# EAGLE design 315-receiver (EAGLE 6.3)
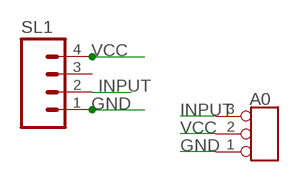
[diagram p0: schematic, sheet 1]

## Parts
A0  TINKER_3P_DIP  [3P_2.0_DIP]
SL1  M04  [4P-NEW]

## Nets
GND: A0.1 SL1.1
INPUT: A0.3 SL1.2
VCC: A0.2 SL1.4
Unconnected: SL1.3

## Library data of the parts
A0 = Connector:TINKER_3P_DIP
SL1 = con-amp-quick:M04: AMP QUICK CONNECTOR

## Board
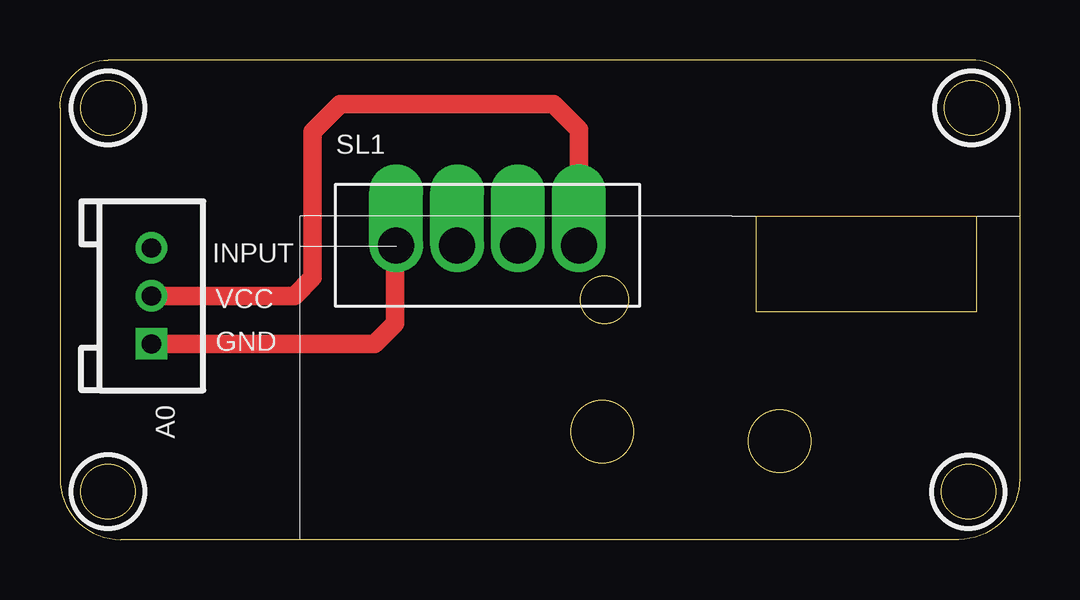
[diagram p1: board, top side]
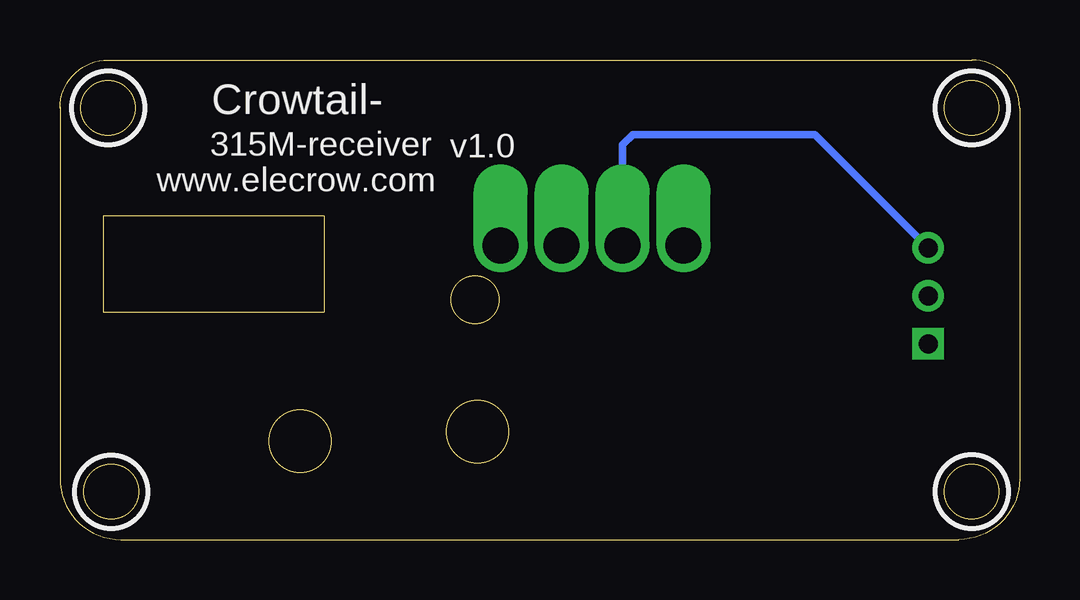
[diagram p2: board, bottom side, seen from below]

Size 40.01 x 20 mm. Coordinates in mm from the lower left corner, seen from the top.
Outline: 40,18 arc90 38,20 2,20 arc90 0,18 0,2.54 arc90 2.54,0 12.32,0
Outline: 40.01,18.03 40.01,2.54 arc-90 37.47,0 10,0
Outline: 29,13.5 29,9.5 38.2,9.5 38.2,13.5 29,13.5
Outline: circle at 2,18 radius 1.14
Outline: circle at 2,2 radius 1.14
Outline: circle at 38,18 radius 1.14
Outline: circle at 22.7,10 radius 1
Outline: circle at 30,4.1 radius 1.3
Outline: circle at 22.6,4.5 radius 1.3
Outline: circle at 37.87,2 radius 1.14
Copper layers (1*16): Top 0.035mm / dielectric 1.5mm / Bottom 0.035mm
Design rules "default *": minimum track width 10mil, minimum drill 24mil, track to track 8mil, track to pad 8mil, pad to pad 8mil, via to via 8mil, smd to smd 8mil, copper to edge 20mil, drill to drill 8mil, minimum pad ring 10mil, minimum via ring 8mil, stop-mask expansion 4mil, vias tented up to drill 0mil, thermal gap 10mil
tRestrict: area 0.5,16.5 to 3.5,19.5; area 0.5,0.5 to 3.5,3.5; area 36.5,16.5 to 39.5,19.5; area 36.3,0.5 to 39.4,3.5
bRestrict: area 0.5,16.5 to 3.5,19.5; area 0.5,0.5 to 3.5,3.5; area 36.5,16.5 to 39.5,19.5; area 36.3,0.5 to 39.4,3.5

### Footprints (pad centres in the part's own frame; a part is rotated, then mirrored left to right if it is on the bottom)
3P_2.0_DIP = drill 0.8 pad 1.27 square: 1 -2,0 | drill 0.8 pad 1.27: 2 0,0; 3 2,0
4P-NEW = drill 1.5 pad 1.676 offset: 1 0,0; 2 2.54,0; 3 5.08,0; 4 7.62,0

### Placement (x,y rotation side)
A0  3.81,10.16 90 top
SL1  14.01,12.27 0 top

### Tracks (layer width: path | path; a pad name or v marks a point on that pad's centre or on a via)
GND
  Top 0.762: A0.1 13.11,8.16 13.97,9.02 13.97,12.23 SL1.1
INPUT
  Bottom 0.305: A0.3 8.54,16.89 16.13,16.89 16.55,16.47 SL1.2
VCC
  Top 0.762: A0.2 9.78,10.16 10.54,10.92 10.54,17.02 11.68,18.16 20.57,18.16 21.63,17.1 SL1.4

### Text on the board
tPlace: INPUT | VCC | GND
bPlace: Crowtail- | v1.0 | 315M-receiver | www.elecrow.com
